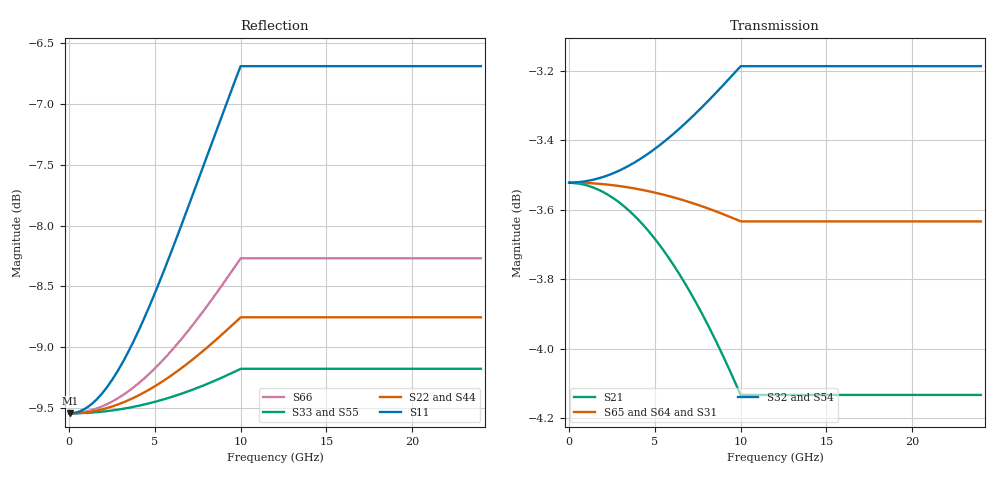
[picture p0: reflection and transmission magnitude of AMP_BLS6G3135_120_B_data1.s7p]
! Created Mon May 10 14:37:55 2010
# ghz S ma R 50
! 7 Port Network Data from SP1.SP block
! freq  magS11  angS11  magS12  angS12  magS13  angS13  magS14  angS14
!  magS15  angS15  magS16  angS16  magS17  angS17
!  magS21  angS21
!  magS22  angS22  magS23  angS23  magS24  angS24  magS25  angS25
!  magS26  angS26  magS27  angS27
!  magS31  angS31  magS32  angS32
!  magS33  angS33  magS34  angS34  magS35  angS35  magS36  angS36
!  magS37  angS37
!  magS41  angS41  magS42  angS42  magS43  angS43
!  magS44  angS44  magS45  angS45  magS46  angS46  magS47  angS47
!  magS51  angS51  magS52  angS52  magS53  angS53  magS54  angS54
!  magS55  angS55  magS56  angS56  magS57  angS57
!  magS61  angS61
!  magS62  angS62  magS63  angS63  magS64  angS64  magS65  angS65
!  magS66  angS66  magS67  angS67
!  magS71  angS71  magS72  angS72
!  magS73  angS73  magS74  angS74  magS75  angS75  magS76  angS76
!  magS77  angS77
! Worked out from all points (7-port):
!   2400 points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, 10 MHz to 24 GHz, reference 50 ohm
!   strongest paths, dB at 10 MHz, 6.01 GHz, 12.01 GHz, 18.01 GHz, 24 GHz:
!     S32: -3.5, -3.4, -3.2, -3.2, -3.2
!     S54: -3.5, -3.5, -3.5, -3.5, -3.5
!     S65: -3.5, -3.6, -3.6, -3.6, -3.6
!     S64: -3.5, -3.6, -3.8, -3.8, -3.8
!     S31: -3.5, -3.7, -4.0, -4.0, -4.0
!     S21: -3.5, -3.8, -4.1, -4.1, -4.1
!   lowest |S11| = -9.5 dB at 70 MHz (marker M1), VSWR 2.00, Z = 25 + j0.193 ohm
!   |S11| at or under -10 dB: nowhere
